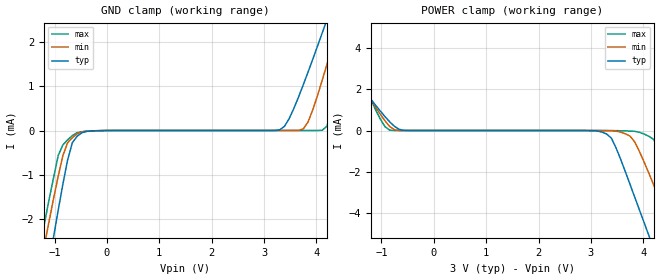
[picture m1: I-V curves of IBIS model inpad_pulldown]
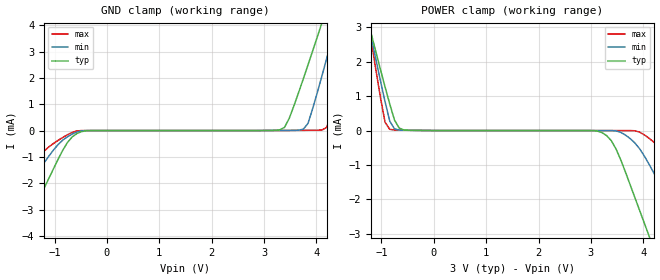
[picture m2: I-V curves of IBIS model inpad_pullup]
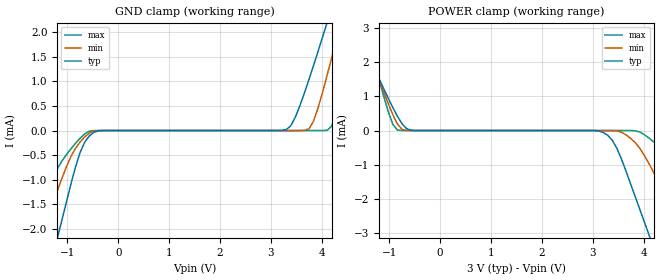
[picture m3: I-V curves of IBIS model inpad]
[IBIS Ver]   2.1
[File Name]   dac2932p.ibs
[File Rev]   1.1
[Source]   Preliminary IBIS Model Generated Manually
[Notes]
   Package information estimated
[Disclaimer]   This information is for modeling purposes only
[Copyright]   (c) 2005, Texas Instruments Inc.
[Component]   TQFP48
[Manufacturer]   Texas Instruments
[Package]
| Variable   Typ   Min   Max
R_pkg   0.1   0.1   0.1
L_pkg   3.0nH   3.0nH   3.0nH
C_pkg   3.0pF   3.0pF   3.0pF
[Pin]   signal_name   model_name   R_pin  L_pin   C_pin
   1   D11   inpad   0.1   3.0nH   3.0pF
   2   D10   inpad   0.1   3.0nH   3.0pF
   3   D9   inpad   0.1   3.0nH   3.0pF
   4   D8   inpad   0.1   3.0nH   3.0pF
   5   D7   inpad   0.1   3.0nH   3.0pF
   6   D6   inpad   0.1   3.0nH   3.0pF
   7   D5   inpad   0.1   3.0nH   3.0pF
   8   D4   inpad   0.1   3.0nH   3.0pF
   9   D3   inpad   0.1   3.0nH   3.0pF
   10   D2   inpad   0.1   3.0nH   3.0pF
   11   D1   inpad   0.1   3.0nH   3.0pF
   12   D0   inpad   0.1   3.0nH   3.0pF
   13   dgnd   GND   0.1   3.0nH   3.0pF
   14   +vd   POWER   0.1   3.0nH   3.0pF
   15   clk   inpad   0.1   3.0nH   3.0pF
   16   pd   inpad_pulldown   0.1   3.0nH   3.0pF
   17   stbyb   inpad_pullup   0.1   3.0nH   3.0pF
   18   csb   inpad_pulldown   0.1   3.0nH   3.0pF
   19   gset   inpad_pulldown   0.1   3.0nH   3.0pF
   20   dgnd   GND   0.1   3.0nH   3.0pF
   21   agnd   GND   0.1   3.0nH   3.0pF
   22   agnd   GND   0.1   3.0nH   3.0pF
|  23   fsa2   0.1   3.0nH   3.0pF
|  24   fsa1   0.1   3.0nH   3.0pF
|  25   refin   0.1   3.0nH   3.0pF
|  26   iout1b   0.1   3.0nH   3.0pF
|  27   iout1   0.1   3.0nH   3.0pF
   28   agnd   GND   0.1   3.0nH   3.0pF
   29   +va   POWER   0.1   3.0nH   3.0pF
   30   +va   POWER   0.1   3.0nH   3.0pF
   31   agnd   GND   0.1   3.0nH   3.0pF
   32   agnd   GND   0.1   3.0nH   3.0pF
|  33   iout2   0.1   3.0nH   3.0pF
|  34   iout2b   0.1   3.0nH   3.0pF
   35   +vav   POWER   0.1   3.0nH   3.0pF
|  36   nc   0.1   3.0nH   3.0pF
|  37   vout1   0.1   3.0nH   3.0pF
|  38   vout2   0.1   3.0nH   3.0pF
|  39   vout3   0.1   3.0nH   3.0pF
|  40   vout4   0.1   3.0nH   3.0pF
   41   agndv   GND   0.1   3.0nH   3.0pF
|  42   refv   0.1   3.0nH   3.0pF
   43   +vdv   POWER   0.1   3.0nH   3.0pF
   44   pdv   inpad_pulldown   0.1   3.0nH   3.0pF
   45   din   inpad   0.1   3.0nH   3.0pF
   46   sclk   inpad   0.1   3.0nH   3.0pF
   47   syncb   inpad   0.1   3.0nH   3.0pF
   48   dgndv   GND   0.1   3.0nH   3.0pF
| End of package information
| Models and submodels in the file (3): inpad_pulldown (Input), inpad_pullup (Input), inpad (Input)
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|   Model inpad_pulldown
[Model]   inpad_pulldown
Model_type   Input
Polarity   Non-Inverting
| signals   A, Y
Vinl = 0.8V
Vinh = 2.4V
|   typ   min   max
C_comp   1.5p   1.5p   1.5p
|   typ   min   max
[Temperature Range]   25   -40.0   90
|   typ   min   max
[Voltage Range]   3.00V   2.70V   3.30V
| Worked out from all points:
|   GND clamp passes 1 mA (typ) near -0.80 V on its own axis
|   POWER clamp passes 1 mA (typ) near -1.04 V on its own axis
[GND_clamp]
|   Voltage   I(typ)   I(min)   I(max)
-3V       -16.11mA   -13.92mA   -14.04mA
-1.29V    -4.291mA   -3.212mA   -2.725mA
-1.11V    -3.048mA   -2.095mA   -1.605mA
-1.02V    -2.427mA   -1.554mA   -1.08mA
-840mV    -1.214mA   -568.6uA   -325.3uA
-570mV    -131.3uA   -76.16uA   -50.47uA
3.3V      17.11uA    1.089uA    1.157uA
3.75V     1.038mA    36.21uA    1.222uA
4.11V     2.207mA    1.135mA    5.972uA
4.38V     3.114mA    2.232mA    853.1uA
4.65V     4.033mA    3.367mA    2.327mA
6V        8.703mA    9.192mA    10.23mA
[POWER_clamp]
|   Voltage   I(typ)   I(min)   I(max)
-3V       7.659mA    9.192mA    12.01mA
-2.28V    5.166mA    6.068mA    7.745mA
-1.83V    3.624mA    4.134mA    5.099mA
-840mV    419.7uA    193.5uA    15.99uA
3.21V     -73.45uA   -5.447uA   877.8nA
3.39V     -365.5uA   -14.65uA   -2.282uA
3.75V     -2.634mA   -277.6uA   -25.33uA
4.02V     -4.499mA   -1.554mA   -176.2uA
4.2V      -5.742mA   -2.649mA   -434.5uA
4.56V     -8.231mA   -4.905mA   -2.533mA
4.92V     -10.72mA   -7.161mA   -4.897mA
6V        -18.18mA   -13.92mA   -12.06mA
|   Model inpad_pullup
[Model]   inpad_pullup
Model_type   Input
Polarity   Non-Inverting
| signals   A, Y
Vinl = 0.8V
Vinh = 2.4V
|   typ   min   max
C_comp   1.5p   1.5p   1.5p
|   typ   min   max
[Temperature Range]   25   -40.0   90
|   typ   min   max
[Voltage Range]   3.00V   2.70V   3.30V
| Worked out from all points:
|   GND clamp passes 1 mA (typ) near -0.91 V on its own axis
|   POWER clamp passes 1 mA (typ) near -0.88 V on its own axis
[GND_clamp]
|   Voltage   I(typ)   I(min)   I(max)
-3V       -9.633mA   -6.448mA   -4.89mA
-2.55V    -7.772mA   -5.142mA   -3.85mA
-2.19V    -6.284mA   -4.098mA   -3.017mA
-1.65V    -4.054mA   -2.532mA   -1.769mA
-660mV    -237.3uA   -131.9uA   -70.08uA
3.39V     118uA      5.286uA    929.7nA
3.84V     2.495mA    272.8uA    9.952uA
4.11V     4.119mA    2.105mA    22.44uA
4.2V      4.666mA    2.762mA    125.2uA
4.38V     5.767mA    4.096mA    1.532mA
4.65V     7.426mA    6.126mA    4.156mA
6V        15.8mA     16.42mA    17.81mA
[POWER_clamp]
|   Voltage   I(typ)   I(min)   I(max)
-3V       13.93mA    16.42mA    20.87mA
-1.29V    3.393mA    3.427mA    3.563mA
-930mV    1.27mA     840.5uA    242.4uA
-840mV    770.4uA    272.8uA    33.72uA
-570mV    16.23uA    9.166uA    10.75uA
3.21V     -58.57uA   -1.019uA   -1.069uA
3.48V     -536.5uA   -11.07uA   -1.069uA
3.93V     -2.321mA   -529.3uA   -47.13uA
4.11V     -3.064mA   -978.4uA   -224.6uA
4.83V     -6.037mA   -3.054mA   -1.493mA
5.46V     -8.64mA    -4.881mA   -2.948mA
6V        -10.87mA   -6.448mA   -4.196mA
|   Model inpad
[Model]   inpad
Model_type   Input
Polarity   Non-Inverting
| signals   A, Y
Vinl = 0.8V
Vinh = 2.4V
|   typ   min   max
C_comp   1.5p   1.5p   1.5p
|   typ   min   max
[Temperature Range]   25   -40.0   90
|   typ   min   max
[Voltage Range]   3.00V   2.70V   3.30V
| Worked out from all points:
|   GND clamp passes 1 mA (typ) near -0.91 V on its own axis
|   POWER clamp passes 1 mA (typ) near -1.04 V on its own axis
[GND_clamp]
|   Voltage   I(typ)   I(min)   I(max)
-3V       -9.632mA   -6.447mA   -4.889mA
-1.83V    -4.796mA   -3.053mA   -2.184mA
-1.47V    -3.31mA    -2.009mA   -1.356mA
-1.2V     -2.196mA   -1.229mA   -781.3uA
-750mV    -444.9uA   -233.9uA   -156.1uA
-570mV    -111.7uA   -51.68uA   -14.4uA
3.3V      16.05uA    51.23pA    6.106pA
3.75V     1.036mA    35.06uA    9.73pA
4.11V     2.205mA    1.134mA    4.672uA
4.38V     3.113mA    2.231mA    851.7uA
4.65V     4.032mA    3.366mA    2.326mA
6V        8.701mA    9.19mA     10.23mA
[POWER_clamp]
|   Voltage   I(typ)   I(min)   I(max)
-3V       7.657mA    9.19mA     12.01mA
-1.65V    3.011mA    3.366mA    4.048mA
-1.47V    2.406mA    2.607mA    3.009mA
-840mV    418.6uA    192.4uA    14.68uA
-570mV    7.829uA    157.8nA    300.4pA
3.21V     -57.57uA   -2.628nA   -3.073pA
3.48V     -535.5uA   -10.06uA   -6.158pA
3.93V     -2.32mA    -528.3uA   -46.06uA
4.11V     -3.063mA   -977.4uA   -223.5uA
4.83V     -6.036mA   -3.053mA   -1.492mA
5.46V     -8.639mA   -4.88mA    -2.947mA
6V        -10.87mA   -6.447mA   -4.195mA
